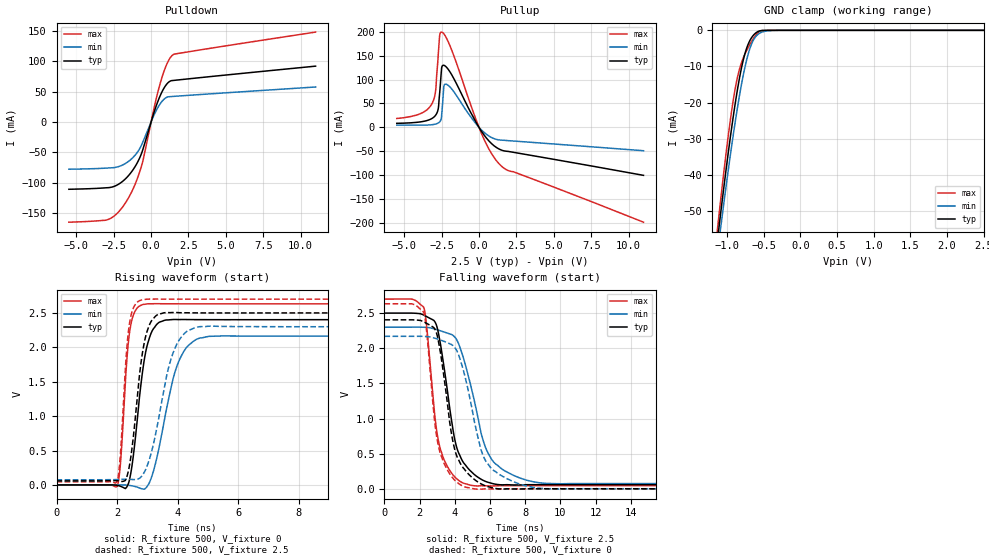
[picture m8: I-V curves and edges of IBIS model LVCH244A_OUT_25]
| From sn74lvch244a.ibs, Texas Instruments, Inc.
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[Model]   LVCH244A_OUT_25
Model_type  3-state
Enable   Active-Low
Vref =   0
Rref =   500
Cref =   30p
Vmeas =   1.25
| variable   typ   min   max
C_comp   5.10pF   4.81pF   5.63pF
| C_pullup   6.78pF   5.69pF   7.38pF
| C_pulldown   6.20pF   4.67pF   7.70pF
| C_tri-state   5.10pF   4.81pF   5.63pF
[Temperature Range]   40   100   -40
| Ambient temperature   25   85   -40
[Voltage range]   2.5   2.3   2.7
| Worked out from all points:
|   slope of the pulldown table from 0 to 0.375 V, typ, clamps not added: 13.1 ohm
|   slope of the pullup table from 0 to 0.375 V, typ, clamps not added: 21.5 ohm
|   GND clamp passes 1 mA (typ) near -0.62 V on its own axis
|   rising waveform, R_fixture 500, V_fixture 0: 20-80 % time 388ps typ, 646ps min, 235ps max; typ from 0 V to 2.4 V
|   falling waveform, R_fixture 500, V_fixture 2.5: 20-80 % time 945ps typ, 1.37ns min, 710ps max; typ from 2.5 V to 0.058 V
|   rising waveform, R_fixture 500, V_fixture 2.5: 20-80 % time 377ps typ, 639ps min, 229ps max; typ from 0.058 V to 2.5 V
|   falling waveform, R_fixture 500, V_fixture 0: 20-80 % time 898ps typ, 1.25ns min, 697ps max; typ from 2.4 V to 0 V
[GND Clamp]
| LVCH244A_OUT_25
|   Voltage   I(typ)   I(min)   I(max)
-5.5V     -943.7mA   -897.4mA   -1.02A
-1.135V   -58.81mA   -62.42mA   -55.76mA
-1.105V   -53.67mA   -57.57mA   -50.2mA
-1.08V    -49.46mA   -53.57mA   -45.65mA
-950mV    -28.86mA   -33.85mA   -24.12mA
-855mV    -16.05mA   -21.05mA   -12.76mA
-785mV    -8.772mA   -13.04mA   -7.971mA
-715mV    -4mA       -6.818mA   -4.874mA
-645mV    -1.466mA   -2.862mA   -2.363mA
-575mV    -299.5uA   -1.059mA   -590.9uA
-295mV    -461nA     -9.889uA   -89.12nA
2.5V      1.156nA    85.59nA    -1.38nA
[Pulldown]
| LVCH244A_OUT_25
|   Voltage   I(typ)   I(min)   I(max)
-5.5V     -110.9mA   -77.86mA   -165.2mA
-2.885V   -108.3mA   -75.88mA   -160.8mA
-2.27V    -103.9mA   -74.19mA   -150.6mA
-1.655V   -92.24mA   -67.45mA   -131mA
-1.125V   -75.68mA   -56.24mA   -105.9mA
-690mV    -54.9mA    -40.56mA   -76.54mA
-520mV    -42.92mA   -31.16mA   -60.99mA
185mV     14.96mA    10.73mA    21.43mA
600mV     42.83mA    29.69mA    62.82mA
1.04V     62.18mA    40.55mA    94.75mA
1.445V    68.32mA    42.07mA    110.4mA
11V       91.99mA    57.64mA    148.1mA
[Pullup]
| LVCH244A_OUT_25
|   Voltage   I(typ)   I(min)   I(max)
-5.5V     8.51mA     4.863mA    18.58mA
-3.91V    11.55mA    4.714mA    28.82mA
-3.14V    18.79mA    5.666mA    49.97mA
-2.905V   25.32mA    6.979mA    75.87mA
-2.73V    38.61mA    9.098mA    150.1mA
-2.625V   74.51mA    11.69mA    193.3mA
-2.475V   127.2mA    34.48mA    198.8mA
-2.35V    129.6mA    86.31mA    195.3mA
-2.145V   124.6mA    89.55mA    184.5mA
185mV     -9.092mA   -6.052mA   -14.17mA
1.465V    -46.97mA   -26.57mA   -79.91mA
11V       -100.1mA   -48.72mA   -197.9mA
[Ramp]
| LVCH244A_OUT_25
| variable   typ   min   max
dV/dt_r   1.47/4.09E-10   1.34/6.90E-10   1.60/2.42E-10
dV/dt_f   1.47/9.91E-10   1.34/1.41E-09   1.59/7.32E-10
R_load = 500
[Rising Waveform]
| LVCH244A_OUT_25
R_fixture =   500
C_fixture =   0
L_fixture =   0
V_fixture =   0
V_fixture_min = 0
V_fixture_max = 0
|   Time   V(typ)   V(min)   V(max)
0s        750.8pV    3.025nV    28.16nV
2.01ns    -7.229mV   -500.7uV   -16.3mV
2.115ns   -20.85mV   -687.4uV   335.9mV
2.305ns   -39.11mV   -2.44mV    1.715V
2.42ns    97.37mV    -8.445mV   2.242V
2.985ns   2.014V     -26.53mV   2.631V
3.35ns    2.351V     468.7mV    2.634V
4.03ns    2.403V     1.79V      2.632V
5.045ns   2.402V     2.159V     2.632V
50ns      2.402V     2.163V     2.632V
[Falling Waveform]
| LVCH244A_OUT_25
R_fixture =   500
C_fixture =   0
L_fixture =   0
V_fixture =   2.5
V_fixture_min = 2.3
V_fixture_max = 2.7
|   Time   V(typ)   V(min)   V(max)
0s        2.5V       2.3V       2.7V
2.23ns    2.473V     2.299V     2.584V
2.89ns    2.367V     2.272V     983.4mV
3.32ns    1.843V     2.237V     459.3mV
4.045ns   649mV      2.146V     157mV
4.925ns   246.4mV    1.45V      49.59mV
5.575ns   124.5mV    718.5mV    43.08mV
6.135ns   74.78mV    403.9mV    40.11mV
8.84ns    58.06mV    83.82mV    44.6mV
50ns      58.46mV    74.07mV    44.5mV
[Rising Waveform]
| LVCH244A_OUT_25
R_fixture =   500
C_fixture =   0
L_fixture =   0
V_fixture =   2.5
V_fixture_min = 2.3
V_fixture_max = 2.7
|   Time   V(typ)   V(min)   V(max)
0s        58.44mV    74mV       44.5mV
2.005ns   60.48mV    78.32mV    52mV
2.105ns   53.81mV    79.81mV    424mV
2.29ns    81.23mV    82.73mV    1.81V
2.4ns     262.7mV    81.43mV    2.32V
2.87ns    2.004V     163.3mV    2.695V
3.165ns   2.404V     530mV      2.701V
3.845ns   2.506V     1.914V     2.7V
4.725ns   2.5V       2.3V       2.7V
50ns      2.5V       2.3V       2.7V
[Falling Waveform]
| LVCH244A_OUT_25
R_fixture =   500
C_fixture =   0
L_fixture =   0
V_fixture =   0
V_fixture_min = 0
V_fixture_max = 0
|   Time   V(typ)   V(min)   V(max)
0s        2.405V     2.17V      2.633V
2.23ns    2.377V     2.169V     2.513V
2.39ns    2.356V     2.167V     2.262V
2.875ns   2.268V     2.142V     911.5mV
3.185ns   1.936V     2.117V     496.2mV
3.935ns   623.2mV    2.028V     138.3mV
4.685ns   234.3mV    1.488V     18.21mV
5.785ns   37.76mV    385.6mV    -1.51mV
8.665ns   -348.3uV   11.26mV    100.4uV
50ns      25.66uV    67.52uV    8.426uV
